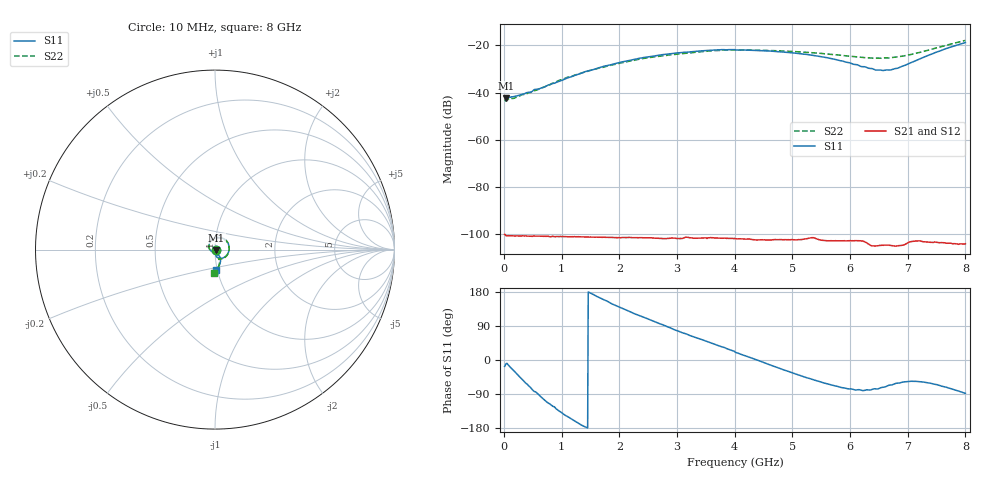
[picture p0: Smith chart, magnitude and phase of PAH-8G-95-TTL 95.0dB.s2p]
! MTS Systemtechnik GmbH
! S-Parameters
! Model: PAH-8G/95-TTL
! Attenuation Step: 95.0dB
! Rohde & Schwarz ZVB8 2Ports - Version 4.11 - 1145.1010k08 SN: 100119
! S2P File Measurements:
! S11 S21 S12 S22
# HZ  S  DB  R  50.00
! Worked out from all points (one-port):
!   800 points, 10 MHz to 8 GHz, reference 50 ohm
!   lowest |S11| = -42.4 dB at 30 MHz (marker M1), VSWR 1.02, Z = 50.7 - j0.144 ohm
!   |S11| at or under -10 dB: start of sweep to end of sweep
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1e7  -41.65 -16.9  -100.21 -2.2  -100.53 0.7  -42.91 -17.0
3e7  -42.43 -10.8  -100.72 -5.1  -100.95 -6.7  -43.55 -12.3
7e7  -42.19 -12.5  -100.77 -10.5  -100.74 -9.9  -42.96 -14.1
1.9e8  -41.58 -31.6  -100.96 -26.8  -100.87 -26.8  -42.20 -34.3
4.5e8  -39.91 -70.8  -100.97 -62.9  -101.05 -62.0  -39.97 -72.9
1.08e9  -33.97 -147.6  -101.18 -148.7  -101.19 -148.7  -33.65 -145.6
1.35e9  -31.63 -172.4  -101.27 174.6  -101.26 174.3  -31.65 -168.5
1.72e9  -28.90 159.7  -101.43 124.0  -101.44 124.3  -29.24 163.5
2.03e9  -27.06 137.6  -101.61 82.0  -101.64 82.2  -27.37 142.1
2.68e9  -24.15 96.7  -101.90 -7.3  -101.86 -7.0  -24.62 102.0
3.43e9  -22.28 53.9  -101.75 -107.9  -101.79 -108.2  -22.63 58.6
3.78e9  -21.76 34.7  -101.88 -156.8  -101.81 -156.4  -22.02 39.8
4.01e9  -21.88 20.3  -102.11 170.2  -102.05 170.3  -21.97 26.4
4.7e9  -22.51 -17.8  -102.39 77.3  -102.45 77.0  -22.22 -9.5
5.34e9  -24.16 -50.9  -101.60 -13.5  -101.65 -13.5  -23.06 -39.2
5.73e9  -25.84 -67.8  -102.97 -68.9  -102.91 -68.7  -23.90 -54.0
6.45e9  -30.44 -76.3  -105.12 -168.8  -105.25 -168.6  -25.36 -67.4
6.67e9  -30.41 -66.8  -104.83 164.7  -104.88 164.7  -25.31 -67.1
6.83e9  -29.61 -61.0  -105.08 148.2  -105.07 148.4  -24.80 -67.3
7.06e9  -27.27 -56.1  -103.27 119.7  -103.26 119.8  -23.81 -67.8
7.63e9  -21.60 -70.3  -103.75 30.3  -103.85 30.0  -20.19 -79.0
8e9  -18.76 -88.1  -104.21 -20.4  -104.48 -20.2  -17.86 -92.8
